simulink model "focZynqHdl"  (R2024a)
settings: Solver=FixedStepDiscrete  StartTime=0.0  StopTime=inf  RelTol=1e-3
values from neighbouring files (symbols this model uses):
  dataRange = Rotor velocity
                        radian/sec
                        800.0
                        -800.0
                    
                
                
                    
                        Phase current
                        Ampere
                        12.0
                        -12.0    [focZynqData.sldd]
  encoder = US Digital E2-1250-197-HI
                0.0
                0
                1250.0
                5000.0
                0.0012566370614359172
                0
                20.0    [focZynqData.sldd]
  paramAdcAmperePerCount = -0.000960526315789474 -0.000968421052631579
                
                    
                        Auto
                        
                        
                        -1.0
                        Simulink
                        Parameter
                        Default    [focZynqData.sldd]
  paramAdcCountAtZeroAmpere = 32600.0 32700.0
                
                    
                        Auto
                        
                        
                        -1.0
                        Simulink
                        Parameter
                        Default
                        
                            
                                0    [focZynqData.sldd]
  paramCurrentControlI = 1774.2
                
                    
                        Auto
                        
                        
                        -1.0
                        Simulink
                        Parameter
                        Default
                        
                            
                                0    [focZynqData.sldd]
  paramCurrentControlP = 1.36193
                
                    
                        Auto
                        
                        
                        -1.0
                        Simulink
                        Parameter
                        Default
                        
                            
                                0    [focZynqData.sldd]
  paramCurrentControlSatVoltage = 13.856406460551021
                
                    
                        Auto
                        
                        
                        -1.0
                        Simulink
                        Parameter
                        Default
                        
                            
                                0    [focZynqData.sldd]
  paramEncoderRotorPositionPerCount = 0.0012566370614359172
                
                    
                        Auto
                        
                        
                        -1.0
                        Simulink
                        Parameter
                        Default
                        
                            
                                0    [focZynqData.sldd]
  paramOverCurrentDuration = 0.05
                
                    
                        Auto
                        
                        
                        -1.0
                        Simulink
                        Parameter
                        Default
                        
                            
                                0    [focZynqData.sldd]
  paramOverCurrentEnable = 0.0
                
                    
                        Auto
                        
                        
                        -1.0
                        Simulink
                        Parameter
                        Default
                        
                            
                                0    [focZynqData.sldd]
  paramOverCurrentLimit = 10.45
                
                    
                        Auto
                        
                        
                        -1.0
                        Simulink
                        Parameter
                        Default
                        
                            
                                0    [focZynqData.sldd]
  paramPwmCompareAtZeroVolt = 500.0
                
                    
                        Auto
                        
                        
                        -1.0
                        Simulink
                        Parameter
                        Default
                        
                            
                                0    [focZynqData.sldd]
  paramPwmCompareMax = 1000.0
                
                    
                        Auto
                        
                        
                        -1.0
                        Simulink
                        Parameter
                        Default
                        
                            
                                0    [focZynqData.sldd]
  paramPwmComparePerVolt = 41.666666666666664
                
                    
                        Auto
                        
                        
                        -1.0
                        Simulink
                        Parameter
                        Default
                        
                            
                                0    [focZynqData.sldd]
  pmsm = Dyno 1: BLY172D-24V-4000 Anaheim Automation
                BLY172D-24V-4000 Anaheim Automation
Phase A leads B leads C for counterclockwise rotation
-----------------------------------------------------
Phase A = Yellow
Phase B = Red
Phase C = Black
                
                    
                        Watt
                        Volt
                        rad/sec    [focZynqData.sldd]
  pwm = 2.0E-8
                4.0E-5
                1000.0
                2000.0
                5.0
                1.0E-7    [focZynqData.sldd]
  sampleTime = 4.0E-5
                0.001
                0.001
                4.0E-5
                2.0E-8
                4.0E-5
                0.001
                2.0E-8
                2.0E-8
                2.0E-8    [focZynqData.sldd]
undefined symbols (not defined in the file or in its folder): hex2dec
libraries: simulink x8
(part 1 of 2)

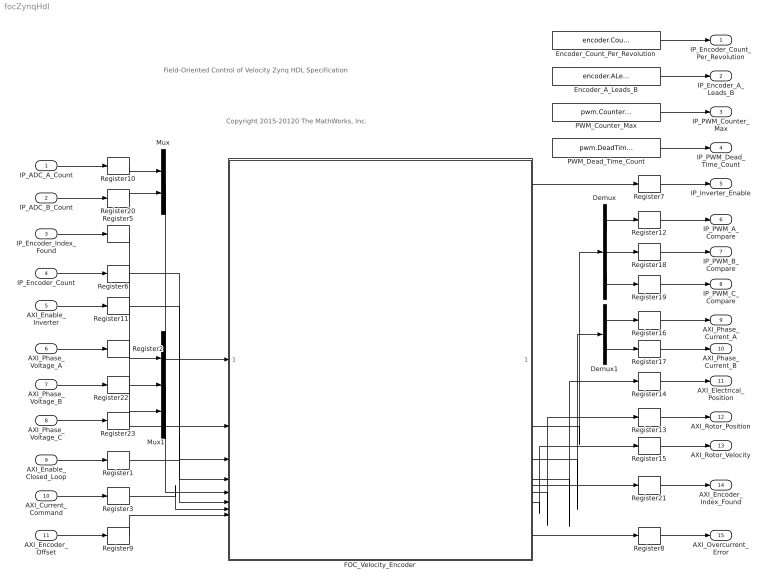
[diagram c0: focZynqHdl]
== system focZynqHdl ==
  note: Field-Oriented Control of Velocity Zynq HDL Specification
  note: Copyright 2015-20120 The MathWorks, Inc.
  IP_ADC_A_Count : Inport  PortDimensions=1  Interpolate=off
  IP_ADC_B_Count : Inport  Port=2  PortDimensions=1  Interpolate=off
  IP_Encoder_Index_Found : Inport  Port=3  Interpolate=off
  IP_Encoder_Count : Inport  Port=4  Interpolate=off
  AXI_Enable_Inverter : Inport  Port=5
  AXI_Phase_Voltage_A : Inport  Port=6
  AXI_Phase_Voltage_B : Inport  Port=7
  AXI_Phase_Voltage_C : Inport  Port=8
  AXI_Enable_Closed_Loop : Inport  Port=9
  AXI_Current_Command : Inport  Port=10
  AXI_Encoder_Offset : Inport  Port=11
  Demux : Demux  Outputs=3
  Demux1 : Demux  Outputs=2
  Encoder_A_Leads_B : Constant  Value=encoder.ALeadsB  OutDataTypeStr=fixdt(0,1,0)  SampleTime=-1
  Encoder_Count_Per_Revolution : Constant  Value=encoder.CountPerRevolution  OutDataTypeStr=fixdt(0,15,0)  SampleTime=-1
  FOC_Velocity_Encoder : Subsystem
  Mux : Mux  Inputs=2
  Mux1 : Mux  Inputs=3
  PWM_Counter_Max : Constant  Value=pwm.CounterMax  OutDataTypeStr=uint16  SampleTime=-1
  PWM_Dead_Time_Count : Constant  Value=pwm.DeadTimeCount  OutDataTypeStr=uint8  SampleTime=-1
  Register{1..3,5..23} (22 alike) : Delay  DelayLength=1
  IP_Encoder_Count_Per_Revolution : Outport  VectorParamsAs1DForOutWhenUnconnected=off
  IP_Encoder_A_Leads_B : Outport  Port=2  VectorParamsAs1DForOutWhenUnconnected=off
  IP_PWM_Counter_Max : Outport  Port=3  VectorParamsAs1DForOutWhenUnconnected=off
  IP_PWM_Dead_Time_Count : Outport  Port=4  VectorParamsAs1DForOutWhenUnconnected=off
  IP_Inverter_Enable : Outport  Port=5  VectorParamsAs1DForOutWhenUnconnected=off
  IP_PWM_A_Compare : Outport  Port=6  VectorParamsAs1DForOutWhenUnconnected=off
  IP_PWM_B_Compare : Outport  Port=7  VectorParamsAs1DForOutWhenUnconnected=off
  IP_PWM_C_Compare : Outport  Port=8  VectorParamsAs1DForOutWhenUnconnected=off
  AXI_Phase_Current_A : Outport  Port=9  VectorParamsAs1DForOutWhenUnconnected=off
  AXI_Phase_Current_B : Outport  Port=10  VectorParamsAs1DForOutWhenUnconnected=off
  AXI_Electrical_Position : Outport  Port=11  VectorParamsAs1DForOutWhenUnconnected=off
  AXI_Rotor_Position : Outport  Port=12  VectorParamsAs1DForOutWhenUnconnected=off
  AXI_Rotor_Velocity : Outport  Port=13  VectorParamsAs1DForOutWhenUnconnected=off
  AXI_Encoder_Index_Found : Outport  Port=14  VectorParamsAs1DForOutWhenUnconnected=off
  AXI_Overcurrent_Error : Outport  Port=15  VectorParamsAs1DForOutWhenUnconnected=off
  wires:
  Demux/2 -> Register18/1
  Demux/3 -> Register19/1
  Demux1/2 -> Register17/1
  IP_ADC_A_Count/1 -> Register10/1
  IP_ADC_B_Count/1 -> Register20/1
  Encoder_Count_Per_Revolution/1 -> IP_Encoder_Count_Per_Revolution/1
  Encoder_A_Leads_B/1 -> IP_Encoder_A_Leads_B/1
  Register15/1 -> AXI_Rotor_Velocity/1
  Register14/1 -> AXI_Electrical_Position/1
  Register13/1 -> AXI_Rotor_Position/1
  Register8/1 -> AXI_Overcurrent_Error/1
  Register7/1 -> IP_Inverter_Enable/1
  IP_Encoder_Count/1 -> Register6/1
  AXI_Current_Command/1 -> Register3/1
  AXI_Phase_Voltage_A/1 -> Register2/1
  AXI_Enable_Closed_Loop/1 -> Register1/1
  Demux/1 -> Register12/1
  Demux1/1 -> Register16/1
  Register16/1 -> AXI_Phase_Current_A/1
  Register17/1 -> AXI_Phase_Current_B/1
  Register12/1 -> IP_PWM_A_Compare/1
  Register18/1 -> IP_PWM_B_Compare/1
  Register19/1 -> IP_PWM_C_Compare/1
  Register10/1 -> Mux/1
  Register20/1 -> Mux/2
  Register5/1 -> FOC_Velocity_Encoder/2(Encoder_Index_Found1)
  IP_Encoder_Index_Found/1 -> Register5/1
  Register1/1 -> FOC_Velocity_Encoder/6(Enable_Current_Control1)
  Mux1/1 -> FOC_Velocity_Encoder/5(Phase_Voltage_Command)
  Register3/1 -> FOC_Velocity_Encoder/7(Current_Command)
  Mux/1 -> FOC_Velocity_Encoder/1(ADC_Phase_Currents)
  Register6/1 -> FOC_Velocity_Encoder/3(Encoder_Count)
  FOC_Velocity_Encoder/3(Phase_Currents) -> Demux1/1
  FOC_Velocity_Encoder/5(Rotor_Position) -> Register13/1
  FOC_Velocity_Encoder/4(Electrical_Position) -> Register14/1
  FOC_Velocity_Encoder/6(Rotor_Velocity) -> Register15/1
  FOC_Velocity_Encoder/2(PWM_Compare) -> Demux/1
  FOC_Velocity_Encoder/8(Error) -> Register8/1
  AXI_Encoder_Offset/1 -> Register9/1
  Register9/1 -> FOC_Velocity_Encoder/8(Encoder_Offset)
  AXI_Enable_Inverter/1 -> Register11/1
  Register11/1 -> FOC_Velocity_Encoder/4(Enable_Inverter_In)
  FOC_Velocity_Encoder/1(Enable_Inverter_Out) -> Register7/1
  Register21/1 -> AXI_Encoder_Index_Found/1
  FOC_Velocity_Encoder/7(Encoder_Index_Found_Out) -> Register21/1
  AXI_Phase_Voltage_B/1 -> Register22/1
  AXI_Phase_Voltage_C/1 -> Register23/1
  Register2/1 -> Mux1/1
  Register22/1 -> Mux1/2
  Register23/1 -> Mux1/3
  PWM_Counter_Max/1 -> IP_PWM_Counter_Max/1
  PWM_Dead_Time_Count/1 -> IP_PWM_Dead_Time_Count/1

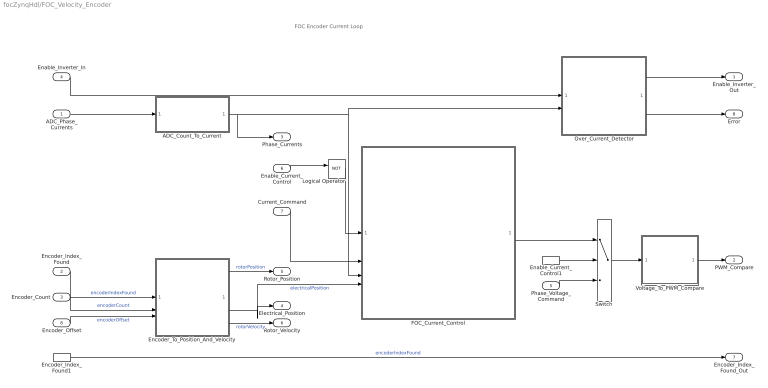
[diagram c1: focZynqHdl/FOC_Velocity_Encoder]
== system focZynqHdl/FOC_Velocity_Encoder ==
  note: FOC Encoder Current Loop
  ADC_Phase_Currents : Inport
  Encoder_Index_Found : Inport  Port=2
  Encoder_Count : Inport  Port=3
  Enable_Inverter_In : Inport  Port=4  OutDataTypeStr=boolean
  Phase_Voltage_Command : Inport  Port=5
  Enable_Current_Control : Inport  Port=6  OutMin=0  OutMax=1  OutDataTypeStr=boolean
  Current_Command : Inport  Port=7
  Encoder_Offset : Inport  Port=8
  ADC_Count_To_Current : Subsystem
  Enable_Current_Control1 : InportShadow  Port=6  OutMin=0  OutMax=1  OutDataTypeStr=boolean
  Encoder_Index_Found1 : InportShadow  Port=2
  Encoder_To_Position_And_Velocity : Subsystem  VariantControl=ctrlVariantPosSns==PosSnsEnum.Encoder
  FOC_Current_Control : Subsystem  Variant=on  VariantControlMode=label  VariantControl=Choice  LabelModeActiveChoice=Default
  Logical Operator : Logic  Operator=NOT  IconShape=distinctive  AllPortsSameDT=off  OutDataTypeStr=boolean
  Over_Current_Detector : Subsystem
  Switch : Switch  Criteria=u2 ~= 0
  Voltage_To_PWM_Compare : Subsystem
  Enable_Inverter_Out : Outport  OutMin=0  OutMax=1  VectorParamsAs1DForOutWhenUnconnected=off
  PWM_Compare : Outport  Port=2  VectorParamsAs1DForOutWhenUnconnected=off
  Phase_Currents : Outport  Port=3  VectorParamsAs1DForOutWhenUnconnected=off
  Electrical_Position : Outport  Port=4  VectorParamsAs1DForOutWhenUnconnected=off
  Rotor_Position : Outport  Port=5  VectorParamsAs1DForOutWhenUnconnected=off
  Rotor_Velocity : Outport  Port=6  VectorParamsAs1DForOutWhenUnconnected=off
  Encoder_Index_Found_Out : Outport  Port=7  OutMin=0  OutMax=1  VectorParamsAs1DForOutWhenUnconnected=off
  Error : Outport  Port=8  OutMin=0  OutMax=1  VectorParamsAs1DForOutWhenUnconnected=off
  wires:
  Encoder_To_Position_And_Velocity/2(Electrical_Position) -> Electrical_Position/1, FOC_Current_Control/4(Electrical_Position)  "electricalPosition"
  Over_Current_Detector/2(Error) -> Error/1
  ADC_Phase_Currents/1 -> ADC_Count_To_Current/1(Count)
  Encoder_Index_Found/1 -> Encoder_To_Position_And_Velocity/1(Index_Found)  "encoderIndexFound"
  Encoder_Count/1 -> Encoder_To_Position_And_Velocity/2(Count)  "encoderCount"
  Encoder_Offset/1 -> Encoder_To_Position_And_Velocity/3(Offset)  "encoderOffset"
  Phase_Voltage_Command/1 -> Switch/3
  ADC_Count_To_Current/1(Current) -> FOC_Current_Control/3(Phase_Current), Over_Current_Detector/2(Phase_Current), Phase_Currents/1
  Encoder_To_Position_And_Velocity/1(Rotor_Position) -> Rotor_Position/1  "rotorPosition"
  Encoder_To_Position_And_Velocity/3(Rotor_Velocity) -> Rotor_Velocity/1  "rotorVelocity"
  Voltage_To_PWM_Compare/1(Compare) -> PWM_Compare/1
  Switch/1 -> Voltage_To_PWM_Compare/1(Voltage)
  Enable_Current_Control/1 -> Logical Operator/1
  Enable_Current_Control1/1 -> Switch/2
  Enable_Inverter_In/1 -> Over_Current_Detector/1(Motor_On)
  Encoder_Index_Found1/1 -> Encoder_Index_Found_Out/1  "encoderIndexFound"
  Over_Current_Detector/1(En_Inv) -> Enable_Inverter_Out/1
  Logical Operator/1 -> FOC_Current_Control/1(Reset)
  Current_Command/1 -> FOC_Current_Control/2(Current_Command)
  FOC_Current_Control/1(Phase_Voltage) -> Switch/1

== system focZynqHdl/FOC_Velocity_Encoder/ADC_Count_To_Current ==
  note: ADC Count to Current
  Count : Inport  OutMin=0  OutMax=2^16-1  OutDataTypeStr=uint16
  Add : Sum  Inputs=+-  OutDataTypeStr=int16
  Bias_To_Remove : Constant  Value=paramAdcCountAtZeroAmpere  OutDataTypeStr=int16  SampleTime=-1
  Data_Type_Convert : DataTypeConversion  OutDataTypeStr=int32
  Product : Product  OutDataTypeStr=fixdt(1,32,19)
  Sat : Saturate  UpperLimit=dataRange.PhaseCurrent.Max  LowerLimit=dataRange.PhaseCurrent.Min  OutDataTypeStr=fixdt(1,16,11)
  Scalar : Constant  Value=paramAdcAmperePerCount  OutDataTypeStr=fixdt(1,16,19)  SampleTime=-1
  Current : Outport  VectorParamsAs1DForOutWhenUnconnected=off
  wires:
  Bias_To_Remove/1 -> Add/2
  Scalar/1 -> Product/2
  Add/1 -> Product/1
  Count/1 -> Data_Type_Convert/1
  Data_Type_Convert/1 -> Add/1
  Product/1 -> Sat/1
  Sat/1 -> Current/1

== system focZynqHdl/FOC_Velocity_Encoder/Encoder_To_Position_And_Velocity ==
  note: Encoder To Position And Velocity
  Index_Found : Inport
  Count : Inport  Port=2  SampleTime=sampleTime.EncoderPosition
  Offset : Inport  Port=3  SampleTime=sampleTime.EncoderPosition
  Encoder_Count_To_Rotor_Position1 : Subsystem
  Rotor_Position_Delta : Subsystem
  Rotor_Position_Delta_To_Velocity : Subsystem  mask(Rotor position delta to velocity){positionDeltaBufferLength=32, sampleFrequency=1/sampleTime.EncoderPosition}
      mask prompts: positionDeltaBufferLength "Delay buffer length (must be power of two)"; sampleFrequency "Sample frequency (Hz)"
      mask help: Calculates velocity by summing the current position delta and a buffer of previous position deltas. Previous position deltas are stored in a circular buffer.
  Rotor_To_Electrical_Position_No_Overflow_Fixpt : Subsystem
  Rotor_Position : Outport  VectorParamsAs1DForOutWhenUnconnected=off
  Electrical_Position : Outport  Port=2  VectorParamsAs1DForOutWhenUnconnected=off
  Rotor_Velocity : Outport  Port=3  VectorParamsAs1DForOutWhenUnconnected=off
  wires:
  Rotor_Position_Delta/1(Position_Delta) -> Rotor_Position_Delta_To_Velocity/1(Position_Delta)  "rotorPositionDelta"
  Rotor_To_Electrical_Position_No_Overflow_Fixpt/1(E) -> Electrical_Position/1
  Count/1 -> Encoder_Count_To_Rotor_Position1/1(Count)
  Index_Found/1 -> Rotor_Position_Delta/3(Encoder_Index_Found)
  Rotor_Position_Delta_To_Velocity/1(Velocity) -> Rotor_Velocity/1
  Encoder_Count_To_Rotor_Position1/1(Position) -> Rotor_Position_Delta/1(Rotor_Position), Rotor_To_Electrical_Position_No_Overflow_Fixpt/1(R), Rotor_Position/1
  Offset/1 -> Rotor_Position_Delta/2(Encoder_Offset), Encoder_Count_To_Rotor_Position1/2(Position_At_Zero_Count)

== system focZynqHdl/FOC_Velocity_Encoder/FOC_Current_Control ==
  Reset : Inport
  Current_Command : Inport  Port=2  OutDataTypeStr=fixdt(1,16,11)
  Phase_Current : Inport  Port=3
  Electrical_Position : Inport  Port=4
  FOC_Current_Control : Subsystem  VariantControl=Default
  FloatingPoint_FOC_Control : Subsystem  VariantControl=Alternative
  Phase_Voltage : Outport

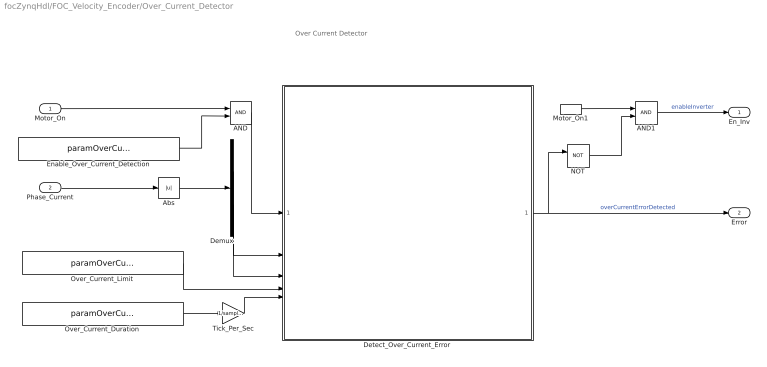
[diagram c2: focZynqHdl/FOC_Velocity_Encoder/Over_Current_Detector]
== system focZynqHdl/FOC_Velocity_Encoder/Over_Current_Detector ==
  note: Over Current Detector
  Motor_On : Inport  OutMin=0  OutMax=1  OutDataTypeStr=boolean
  Phase_Current : Inport  Port=2  OutMin=dataRange.PhaseCurrent.Min  OutMax=dataRange.PhaseCurrent.Max  OutDataTypeStr=fixdt(1,16,11)
  AND : Logic  IconShape=distinctive  AllPortsSameDT=off  OutDataTypeStr=boolean
  AND1 : Logic  IconShape=distinctive  AllPortsSameDT=off  OutDataTypeStr=boolean
  Abs : Abs
  Demux : Demux  Outputs=2
  Detect_Over_Current_Error : Stateflow chart  TreatAsAtomicUnit=on
  Enable_Over_Current_Detection : Constant  Value=paramOverCurrentEnable  OutDataTypeStr=boolean  SampleTime=-1
  Motor_On1 : InportShadow  OutMin=0  OutMax=1  OutDataTypeStr=boolean
  NOT : Logic  Operator=NOT  IconShape=distinctive  AllPortsSameDT=off  OutDataTypeStr=boolean
  Over_Current_Duration : Constant  Value=paramOverCurrentDuration  OutDataTypeStr=fixdt(1,16,14)  SampleTime=-1
  Over_Current_Limit : Constant  Value=paramOverCurrentLimit  OutDataTypeStr=fixdt(1,16,11)  SampleTime=-1
  Tick_Per_Sec : Gain  Gain=1/sampleTime.OverCurrentDetector  ParamDataTypeStr=fixdt(1,16,0)  OutDataTypeStr=uint16
  En_Inv : Outport  VectorParamsAs1DForOutWhenUnconnected=off
  Error : Outport  Port=2  VectorParamsAs1DForOutWhenUnconnected=off
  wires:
  Tick_Per_Sec/1 -> Detect_Over_Current_Error/5(overCurrentDurationTicks)
  Phase_Current/1 -> Abs/1
  Abs/1 -> Demux/1
  Demux/2 -> Detect_Over_Current_Error/3(phaseCurrentB)
  Detect_Over_Current_Error/1(error) -> Error/1, NOT/1  "overCurrentErrorDetected"
  Over_Current_Duration/1 -> Tick_Per_Sec/1
  Over_Current_Limit/1 -> Detect_Over_Current_Error/4(overCurrentLimit)
  Demux/1 -> Detect_Over_Current_Error/2(phaseCurrentA)
  Motor_On/1 -> AND/1
  AND1/1 -> En_Inv/1  "enableInverter"
  NOT/1 -> AND1/2
  Motor_On1/1 -> AND1/1
  AND/1 -> Detect_Over_Current_Error/1(enableOverCurrentDetect)
  Enable_Over_Current_Detection/1 -> AND/2

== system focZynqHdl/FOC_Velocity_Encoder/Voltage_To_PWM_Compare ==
  note: Voltage To PWM Compare
  Voltage : Inport  OutMin=dataRange.PhaseVoltage.Min  OutMax=dataRange.PhaseVoltage.Max  OutDataTypeStr=fixdt(1,16,11)
  Add : Sum  OutDataTypeStr=fixdt(1,32,17)
  Bias : Constant  Value=paramPwmCompareAtZeroVolt  OutDataTypeStr=fixdt(1,16,2)  SampleTime=-1
  Data_Type_Conversion : DataTypeConversion  OutDataTypeStr=uint16
  Saturation : Saturate  UpperLimit=paramPwmCompareMax  LowerLimit=0
  Slope : Gain  Gain=paramPwmComparePerVolt  ParamDataTypeStr=fixdt(1,16,6)  OutDataTypeStr=fixdt(1,32,18)
  Compare : Outport  VectorParamsAs1DForOutWhenUnconnected=off
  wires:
  Data_Type_Conversion/1 -> Compare/1  "pwmCompare"
  Voltage/1 -> Slope/1  "phaseVoltage"
  Slope/1 -> Add/1
  Saturation/1 -> Data_Type_Conversion/1
  Bias/1 -> Add/2
  Add/1 -> Saturation/1

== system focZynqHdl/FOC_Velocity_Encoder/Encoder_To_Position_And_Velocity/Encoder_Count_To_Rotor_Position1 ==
  note: Encoder Count To Rotor Position
  Count : Inport  OutMin=dataRange.EncoderCount.Min  OutMax=dataRange.EncoderCount.Max  OutDataTypeStr=fixdt(0,16,0)
  Position_At_Zero_Count : Inport  Port=2  OutMin=-2*pi  OutMax=2*pi  OutDataTypeStr=fixdt(1,16,12)
  Add : Sum  OutDataTypeStr=fixdt(1,32,27)
  Data_Type_Convert : DataTypeConversion  OutDataTypeStr=fixdt(1,16,12)  RndMeth=Simplest
  Mod_Two_Pi_Once : Subsystem
  Rotor_Position_Per_Count : Gain  Gain=paramEncoderRotorPositionPerCount  ParamDataTypeStr=fixdt(1,16,22)  OutDataTypeStr=fixdt(1,32,25)
  Position : Outport  VectorParamsAs1DForOutWhenUnconnected=off
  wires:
  Count/1 -> Rotor_Position_Per_Count/1
  Position_At_Zero_Count/1 -> Add/2
  Rotor_Position_Per_Count/1 -> Add/1
  Add/1 -> Mod_Two_Pi_Once/1(X)
  Mod_Two_Pi_Once/1(Mod_X_Two_Pi) -> Data_Type_Convert/1  "rotorPosition"
  Data_Type_Convert/1 -> Position/1

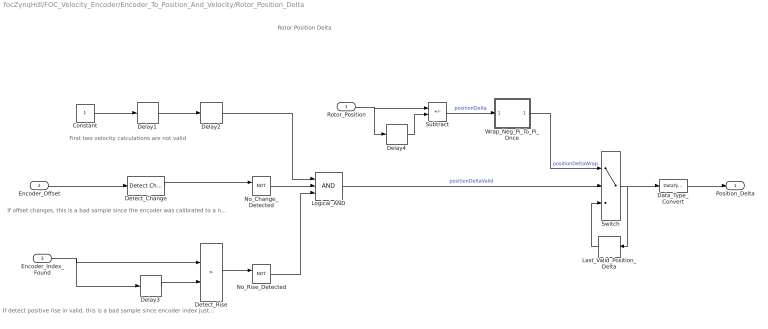
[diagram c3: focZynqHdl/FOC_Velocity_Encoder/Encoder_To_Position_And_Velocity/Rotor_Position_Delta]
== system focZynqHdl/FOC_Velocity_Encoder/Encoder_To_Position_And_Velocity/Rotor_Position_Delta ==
  note: Rotor Position Delta
  note: If detect positive rise in valid, this is a bad sample since encoder index just reset
  note: First two velocity calculations are not valid
  note: If offset changes, this is a bad sample since the encoder was calibrated to a new value
  Rotor_Position : Inport  OutMin=0  OutMax=2*pi  OutDataTypeStr=fixdt(1,16,12)  SampleTime=sampleTime.EncoderPosition
  Encoder_Offset : Inport  Port=2  OutMin=-2*pi  OutMax=2*pi  OutDataTypeStr=fixdt(1,16,12)  SampleTime=sampleTime.EncoderPosition
  Encoder_Index_Found : Inport  Port=3  OutDataTypeStr=boolean  SampleTime=sampleTime.EncoderPosition
  Constant : Constant  OutDataTypeStr=fixdt(1,16,14)  SampleTime=-1
  Data_Type_Convert : DataTypeConversion  OutDataTypeStr=fixdt(1,16,13)  RndMeth=Simplest
  Delay{1..4} (4 alike) : Delay  DelayLength=1
  Detect_Change : simulink/Logic and Bit Operations/Detect Change  vinit=0  OutDataTypeStr=boolean
  Detect_Rise : RelationalOperator  Operator=>  OutDataTypeStr=boolean  ZeroCross=off
  Last_Valid_Position_Delta : Delay  DelayLength=1
  Logical_AND : Logic  Inputs=3  IconShape=distinctive  AllPortsSameDT=off  OutDataTypeStr=boolean
  No_Change_Detected : Logic  Operator=NOT  IconShape=distinctive  AllPortsSameDT=off  OutDataTypeStr=boolean
  No_Rise_Detected : Logic  Operator=NOT  IconShape=distinctive  AllPortsSameDT=off  OutDataTypeStr=boolean
  Subtract : Sum  Inputs=+-  OutDataTypeStr=fixdt(1,32,27)  InputSameDT=on
  Switch : Switch  Criteria=u2 ~= 0  OutDataTypeStr=fixdt(1,32,29)
  Wrap_Neg_Pi_To_Pi_Once : Subsystem
  Position_Delta : Outport  SampleTime=sampleTime.EncoderPosition  VectorParamsAs1DForOutWhenUnconnected=off
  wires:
  Delay1/1 -> Delay2/1
  Constant/1 -> Delay1/1
  Switch/1 -> Last_Valid_Position_Delta/1, Data_Type_Convert/1
  No_Rise_Detected/1 -> Logical_AND/3
  Detect_Rise/1 -> No_Rise_Detected/1
  Last_Valid_Position_Delta/1 -> Switch/3
  Delay3/1 -> Detect_Rise/2
  Logical_AND/1 -> Switch/2  "positionDeltaValid"
  Delay4/1 -> Subtract/2
  Delay2/1 -> Logical_AND/1
  Subtract/1 -> Wrap_Neg_Pi_To_Pi_Once/1(Position)  "positionDelta"
  Rotor_Position/1 -> Delay4/1, Subtract/1
  Encoder_Index_Found/1 -> Delay3/1, Detect_Rise/1
  Wrap_Neg_Pi_To_Pi_Once/1(Wrap) -> Switch/1  "positionDeltaWrap"
  Encoder_Offset/1 -> Detect_Change/1
  Detect_Change/1 -> No_Change_Detected/1
  No_Change_Detected/1 -> Logical_AND/2
  Data_Type_Convert/1 -> Position_Delta/1

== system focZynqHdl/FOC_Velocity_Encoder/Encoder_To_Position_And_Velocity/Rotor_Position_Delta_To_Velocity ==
  note: Rotor Position Delta To Velocity
  Position_Delta : Inport  OutMin=-pi  OutMax=pi  OutDataTypeStr=fixdt(1,16,13)  SampleTime=sampleTime.EncoderPosition
  Rotor_Position_Delta_To_Velocity : MATLAB Function  TreatAsAtomicUnit=on
  Velocity : Outport  SampleTime=sampleTime.EncoderPosition  VectorParamsAs1DForOutWhenUnconnected=off
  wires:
  Position_Delta/1 -> Rotor_Position_Delta_To_Velocity/1(positionDelta)
  Rotor_Position_Delta_To_Velocity/1(rotorVelocity) -> Velocity/1

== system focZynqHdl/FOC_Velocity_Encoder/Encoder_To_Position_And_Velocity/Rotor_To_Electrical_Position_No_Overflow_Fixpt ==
  note: Rotor To Electrical Position
  note: Fixed-point implementation which avoids overflow
  R : Inport  OutDataTypeStr=fixdt(1,16,12)
  Extract_Lower_Bits1 : simulink/Logic and Bit Operations/Bitwise Operator  logicop=AND  UseBitMask=on  BitMask=hex2dec('FFFF')  BitMaskRealWorld=Stored Integer
  Extract_Lower_Bits2 : simulink/Logic and Bit Operations/Bitwise Operator  logicop=AND  UseBitMask=on  BitMask=hex2dec('FFFF')  BitMaskRealWorld=Stored Integer
  Input_Range : SignalSpecification  OutMin=0  OutMax=2*pi
  Normalize : Gain  Gain=1/(2*pi)  ParamDataTypeStr=fixdt(0,16,18)  OutDataTypeStr=fixdt(0,32,16, 'DataTypeOverride', 'Off')
  Pole_Pair_Gain : Gain  Gain=pmsm.PolePairs  ParamDataTypeStr=uint16  OutDataTypeStr=fixdt('uint32', 'DataTypeOverride', 'Off')
  Scale_To_Two_Pi : Gain  Gain=2*pi  ParamDataTypeStr=fixdt(0,16,13)  OutDataTypeStr=fixdt(0,16,12)
  Signed_Fixpt : DataTypeConversion  OutDataTypeStr=fixdt(1,16,12)  ConvertRealWorld=Stored Integer (SI)
  Unsigned_Fixpt : DataTypeConversion  OutDataTypeStr=fixdt(0,16,16, 'DataTypeOverride', 'Off')  ConvertRealWorld=Stored Integer (SI)
  Unsigned_Integer : DataTypeConversion  OutDataTypeStr=fixdt('uint16', 'DataTypeOverride', 'Off')  ConvertRealWorld=Stored Integer (SI)
  E : Outport  VectorParamsAs1DForOutWhenUnconnected=off
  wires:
  R/1 -> Input_Range/1
  Unsigned_Integer/1 -> Pole_Pair_Gain/1
  Pole_Pair_Gain/1 -> Extract_Lower_Bits2/1
  Normalize/1 -> Extract_Lower_Bits1/1
  Extract_Lower_Bits2/1 -> Unsigned_Fixpt/1
  Scale_To_Two_Pi/1 -> Signed_Fixpt/1
  Unsigned_Fixpt/1 -> Scale_To_Two_Pi/1
  Signed_Fixpt/1 -> E/1
  Input_Range/1 -> Normalize/1
  Extract_Lower_Bits1/1 -> Unsigned_Integer/1

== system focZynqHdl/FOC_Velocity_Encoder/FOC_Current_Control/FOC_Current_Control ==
  note: FOC Current Control
  Reset : Inport  SampleTime=sampleTime.CurrentControl
  Current_Command : Inport  Port=2  OutMin=dataRange.PhaseCurrent.Min  OutMax=dataRange.PhaseCurrent.Max  OutDataTypeStr=fixdt(1,16,11)  SampleTime=sampleTime.CurrentControl
  Phase_Current : Inport  Port=3  OutMin=dataRange.PhaseCurrent.Min  OutMax=dataRange.PhaseCurrent.Max  OutDataTypeStr=fixdt(1,16,11)  SampleTime=sampleTime.CurrentControl
  Electrical_Position : Inport  Port=4  OutMin=0  OutMax=2*pi  OutDataTypeStr=fixdt(1,16,12)  SampleTime=sampleTime.CurrentControl
  Clarke_Transform : Subsystem
  DQ_Current_Control : Subsystem
  Inverse_Clarke_Transform : Subsystem  VariantControl=INVERSE_CLARKE_TRANSFORM
  Inverse_Park_Transform : Subsystem
  Park_Transform : Subsystem
  Sat : Saturate  UpperLimit=dataRange.PhaseVoltage.Max  LowerLimit=dataRange.PhaseVoltage.Min  OutDataTypeStr=fixdt(1,16,11)
  Sine_Cosine : Subsystem
  Space_Vector_Modulation : Subsystem  VariantControl=SpaceVectorModulation_JB
  Phase_Voltage : Outport  SampleTime=sampleTime.CurrentControl  VectorParamsAs1DForOutWhenUnconnected=off
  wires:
  Sine_Cosine/1(Sin) -> Park_Transform/3(Sin_Coefficient1), Inverse_Park_Transform/3(Sin_Coefficient1)  "sinCoefficient"
  Sine_Cosine/2(Cos) -> Park_Transform/4(Cos_Coefficient1), Inverse_Park_Transform/4(Cos_Coefficient1)  "cosCoefficient"
  Inverse_Clarke_Transform/1(ABC) -> Space_Vector_Modulation/1(ABC)  "abcVoltage"
  Electrical_Position/1 -> Sine_Cosine/1(P)
  Phase_Current/1 -> Clarke_Transform/1(ABC)
  Clarke_Transform/1(Alpha) -> Park_Transform/1(Alpha)  "alphaCurrent"
  Clarke_Transform/2(Beta) -> Park_Transform/2(Beta1)  "betaCurrent"
  Inverse_Park_Transform/1(Alpha) -> Inverse_Clarke_Transform/1(Alpha)  "alphaVoltage"
  Inverse_Park_Transform/2(Beta) -> Inverse_Clarke_Transform/2(Beta)  "betaVoltage"
  Park_Transform/1(D) -> DQ_Current_Control/3(D_Current)  "dCurrent"
  Park_Transform/2(Q) -> DQ_Current_Control/4(Q_Current)  "qCurrent"
  Current_Command/1 -> DQ_Current_Control/2(Q_Command)
  DQ_Current_Control/1(D_Voltage) -> Inverse_Park_Transform/1(D)  "dVoltage"
  DQ_Current_Control/2(Q_Voltage) -> Inverse_Park_Transform/2(Q)  "qVoltage"
  Space_Vector_Modulation/1(ABC_SVM) -> Sat/1  "svmVoltage"
  Sat/1 -> Phase_Voltage/1
  Reset/1 -> DQ_Current_Control/1(Reset)

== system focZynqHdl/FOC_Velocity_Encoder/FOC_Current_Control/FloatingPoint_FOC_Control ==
  note: FOC Encoder Current Loop current control floating-point algorithm
  Reset : Inport
  Current_Command : Inport  Port=2
  Phase_Current : Inport  Port=3
  Electrical_Position : Inport  Port=4
  Data Type Conversion1 : DataTypeConversion  OutDataTypeStr=single  RndMeth=Nearest
  Data Type Conversion2 : DataTypeConversion  OutDataTypeStr=single  RndMeth=Nearest
  Data Type Conversion3 : DataTypeConversion  OutDataTypeStr=single  RndMeth=Nearest
  Data Type Conversion4 : DataTypeConversion  OutDataTypeStr=fixdt(1,16,11)  RndMeth=Nearest
  FOC_Current_Control : Subsystem
  Phase_Voltage : Outport  VectorParamsAs1DForOutWhenUnconnected=off
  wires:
  Current_Command/1 -> Data Type Conversion1/1
  Data Type Conversion3/1 -> FOC_Current_Control/4(Electrical_Position)
  FOC_Current_Control/1(Phase_Voltage) -> Data Type Conversion4/1
  Reset/1 -> FOC_Current_Control/1(Reset)
  Data Type Conversion1/1 -> FOC_Current_Control/2(Current_Command)
  Data Type Conversion2/1 -> FOC_Current_Control/3(Phase_Current)
  Electrical_Position/1 -> Data Type Conversion3/1
  Phase_Current/1 -> Data Type Conversion2/1
  Data Type Conversion4/1 -> Phase_Voltage/1

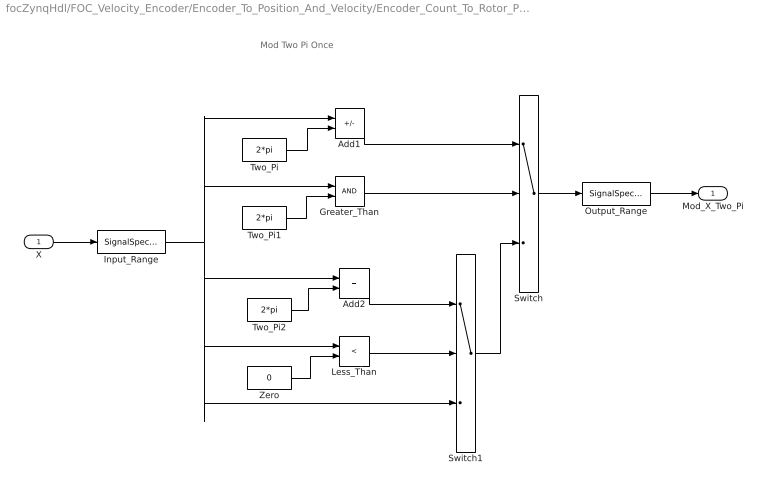
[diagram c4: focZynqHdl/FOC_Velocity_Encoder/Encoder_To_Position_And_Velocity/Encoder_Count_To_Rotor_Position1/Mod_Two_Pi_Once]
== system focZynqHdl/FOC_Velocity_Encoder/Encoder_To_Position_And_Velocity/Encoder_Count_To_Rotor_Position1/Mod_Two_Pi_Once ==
  note: Mod Two Pi Once
  X : Inport
  Add1 : Sum  Inputs=+-  OutDataTypeStr=fixdt(1,32,28)
  Add2 : Sum  OutDataTypeStr=fixdt(1,32,27)
  Greater_Than : RelationalOperator  OutDataTypeStr=boolean
  Input_Range : SignalSpecification  OutMin=-4*pi  OutMax=4*pi
  Less_Than : RelationalOperator  Operator=<  OutDataTypeStr=boolean
  Output_Range : SignalSpecification  OutMin=0  OutMax=2*pi
  Switch : Switch  Criteria=u2 ~= 0  OutDataTypeStr=fixdt(1,32,28)
  Switch1 : Switch  Criteria=u2 ~= 0  OutDataTypeStr=fixdt(1,32,28)
  Two_Pi : Constant  Value=2*pi  OutDataTypeStr=fixdt(1,16,12)  SampleTime=-1
  Two_Pi1 : Constant  Value=2*pi  OutDataTypeStr=fixdt(1,16,12)  SampleTime=-1
  Two_Pi2 : Constant  Value=2*pi  OutDataTypeStr=fixdt(1,16,12)  SampleTime=-1
  Zero : Constant  Value=0  OutDataTypeStr=fixdt(1,16,0)  SampleTime=-1
  Mod_X_Two_Pi : Outport  VectorParamsAs1DForOutWhenUnconnected=off
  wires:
  Input_Range/1 -> Switch1/3, Less_Than/1, Add2/1, Greater_Than/1, Add1/1
  Switch/1 -> Output_Range/1
  X/1 -> Input_Range/1
  Greater_Than/1 -> Switch/2
  Add1/1 -> Switch/1
  Two_Pi/1 -> Add1/2
  Two_Pi1/1 -> Greater_Than/2
  Switch1/1 -> Switch/3
  Less_Than/1 -> Switch1/2
  Add2/1 -> Switch1/1
  Two_Pi2/1 -> Add2/2
  Zero/1 -> Less_Than/2
  Output_Range/1 -> Mod_X_Two_Pi/1

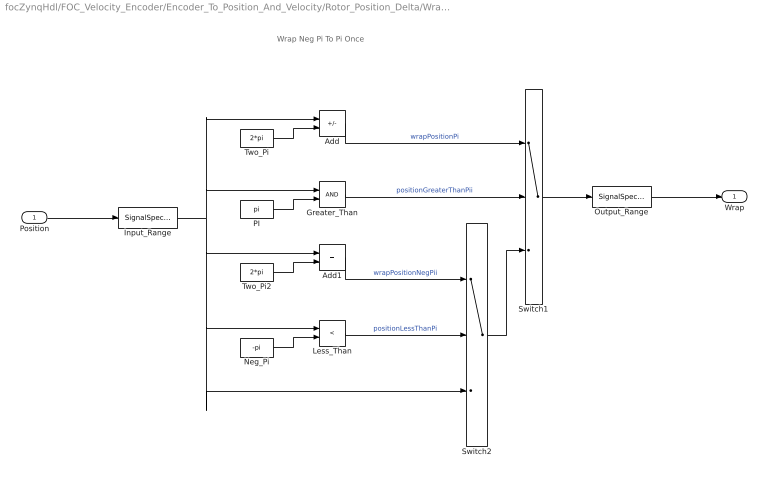
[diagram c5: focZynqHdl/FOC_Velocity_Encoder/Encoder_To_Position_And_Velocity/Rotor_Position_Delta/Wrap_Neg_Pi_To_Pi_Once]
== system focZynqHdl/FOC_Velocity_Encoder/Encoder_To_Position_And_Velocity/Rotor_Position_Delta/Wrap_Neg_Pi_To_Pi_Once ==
  note: Wrap Neg Pi To Pi Once
  Position : Inport
  Add : Sum  Inputs=+-  OutDataTypeStr=fixdt(1,32,29)
  Add1 : Sum  OutDataTypeStr=fixdt(1,32,29)
  Greater_Than : RelationalOperator  OutDataTypeStr=boolean
  Input_Range : SignalSpecification  OutMin=-4*pi  OutMax=4*pi
  Less_Than : RelationalOperator  Operator=<  OutDataTypeStr=boolean
  Neg_Pi : Constant  Value=-pi  OutDataTypeStr=fixdt(1,16,13)  SampleTime=-1
  Output_Range : SignalSpecification  OutMin=-pi  OutMax=pi
  PI : Constant  Value=pi  OutDataTypeStr=fixdt(1,16,13)  SampleTime=-1
  Switch1 : Switch  Criteria=u2 ~= 0  OutDataTypeStr=fixdt(1,32,29)
  Switch2 : Switch  Criteria=u2 ~= 0  OutDataTypeStr=fixdt(1,32,29)
  Two_Pi : Constant  Value=2*pi  OutDataTypeStr=fixdt(1,16,12)  SampleTime=-1
  Two_Pi2 : Constant  Value=2*pi  OutDataTypeStr=fixdt(1,16,12)  SampleTime=-1
  Wrap : Outport  VectorParamsAs1DForOutWhenUnconnected=off
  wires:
  Position/1 -> Input_Range/1
  PI/1 -> Greater_Than/2
  Neg_Pi/1 -> Less_Than/2
  Greater_Than/1 -> Switch1/2  "positionGreaterThanPii"
  Two_Pi/1 -> Add/2
  Add/1 -> Switch1/1  "wrapPositionPi"
  Less_Than/1 -> Switch2/2  "positionLessThanPi"
  Switch2/1 -> Switch1/3
  Two_Pi2/1 -> Add1/2
  Add1/1 -> Switch2/1  "wrapPositionNegPii"
  Switch1/1 -> Output_Range/1
  Output_Range/1 -> Wrap/1
  Input_Range/1 -> Less_Than/1, Switch2/3, Add1/1, Add/1, Greater_Than/1

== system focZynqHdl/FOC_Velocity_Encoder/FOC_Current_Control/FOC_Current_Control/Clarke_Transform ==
  note: Clarke Transform
  note: Converts balanced three-phase quantities into balanced two-phase quantities. The A and B phases are converted to the direct axis (alpha) component and the quadrature axis (beta) component. The alpha and beta components are still dependent on time and speed.
  ABC : Inport
  A : Selector  IndexMode=Zero-based  InputPortWidth=2  IndexOptions=Index vector (dialog)  Indices=0  OutputSizes=1
  Add : Sum  OutDataTypeStr=fixdt(1,16,10)
  Alpha_Gain : Gain  Gain=1/sqrt(3)  ParamDataTypeStr=fixdt(1,16,15)  OutDataTypeStr=fixdt(1,32,28)
  B : Selector  IndexMode=Zero-based  InputPortWidth=2  IndexOptions=Index vector (dialog)  Indices=1  OutputSizes=1
  Beta_Gain : Gain  Gain=2/sqrt(3)  ParamDataTypeStr=fixdt(1,16,14)  OutDataTypeStr=fixdt(1,32,27)
  Alpha : Outport  VectorParamsAs1DForOutWhenUnconnected=off
  Beta : Outport  Port=2  VectorParamsAs1DForOutWhenUnconnected=off
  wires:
  Add/1 -> Beta/1
  B/1 -> Beta_Gain/1
  Beta_Gain/1 -> Add/2
  ABC/1 -> A/1, B/1
  Alpha_Gain/1 -> Add/1
  A/1 -> Alpha_Gain/1, Alpha/1

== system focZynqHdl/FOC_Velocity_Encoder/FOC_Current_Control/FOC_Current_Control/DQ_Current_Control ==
  note: DQ Current Control
  Reset : Inport
  Q_Command : Inport  Port=2  SampleTime=sampleTime.CurrentControl
  D_Current : Inport  Port=3
  Q_Current : Inport  Port=4
  D_Command : Constant  Value=0  OutDataTypeStr=fixdt(1,16,0)  SampleTime=-1
  D_Current_Control : Subsystem
  Q_Current_Control : Subsystem
  Reset1 : InportShadow
  D_Voltage : Outport  VectorParamsAs1DForOutWhenUnconnected=off
  Q_Voltage : Outport  Port=2  VectorParamsAs1DForOutWhenUnconnected=off
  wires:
  Q_Current_Control/1(Voltage) -> Q_Voltage/1
  D_Current_Control/1(Voltage) -> D_Voltage/1
  D_Command/1 -> D_Current_Control/2(Current_Command)
  Q_Command/1 -> Q_Current_Control/2(Current_Command)
  Q_Current/1 -> Q_Current_Control/3(Current_Measured)
  D_Current/1 -> D_Current_Control/3(Current_Measured)
  Reset/1 -> D_Current_Control/1(Reset)
  Reset1/1 -> Q_Current_Control/1(Reset)

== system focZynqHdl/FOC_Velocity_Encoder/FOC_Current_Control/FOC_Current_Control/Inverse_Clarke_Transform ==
  note: Inverse Clarke Transform
  note: Converts direct axis (alpha) component and the quadrature axis (beta) component to balanced three-phase quantities The alpha and beta components are dependent on time and speed.
  Alpha : Inport
  Beta : Inport  Port=2
  Add : Sum  Inputs=-+  OutDataTypeStr=fixdt(1,32,25)
  Add1 : Sum  Inputs=--  OutDataTypeStr=fixdt(1,32,25)
  Data_Type_Convert : DataTypeConversion  OutDataTypeStr=fixdt(1,32,25)  RndMeth=Simplest
  Gain : Gain  Gain=1/2  ParamDataTypeStr=fixdt(1,16,15)  OutDataTypeStr=fixdt(1,32,27)
  Gain1 : Gain  Gain=sqrt(3)/2  ParamDataTypeStr=fixdt(1,16,15)  OutDataTypeStr=fixdt(1,32,26)
  Mux : Mux  Inputs=3
  ABC : Outport  VectorParamsAs1DForOutWhenUnconnected=off
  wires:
  Gain/1 -> Add1/1, Add/1
  Gain1/1 -> Add1/2, Add/2
  Add/1 -> Mux/2
  Add1/1 -> Mux/3
  Beta/1 -> Gain1/1
  Alpha/1 -> Gain/1, Data_Type_Convert/1
  Mux/1 -> ABC/1
  Data_Type_Convert/1 -> Mux/1

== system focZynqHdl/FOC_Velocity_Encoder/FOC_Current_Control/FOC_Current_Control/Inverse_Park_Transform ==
  note: Inverse Park Transform
  note: Converts orthogonal rotating reference frame (dq) to two-phase orthogonal stationary reference frame (alpha, beta)
  D : Inport
  Q : Inport  Port=2
  Sin_Coefficient : Inport  Port=3
  Cos_Coefficient : Inport  Port=4
  Add1 : Sum  Inputs=+-  OutDataTypeStr=fixdt(1,16,10)
  Add2 : Sum  OutDataTypeStr=fixdt(1,16,10)
  Cos_Coefficient1 : InportShadow  Port=4
  Product{1..4} (4 alike) : Product  OutDataTypeStr=fixdt(1,32,27)  RndMeth=Simplest
  Sin_Coefficient1 : InportShadow  Port=3
  Alpha : Outport  VectorParamsAs1DForOutWhenUnconnected=off
  Beta : Outport  Port=2  VectorParamsAs1DForOutWhenUnconnected=off
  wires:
  Add2/1 -> Beta/1
  Add1/1 -> Alpha/1
  Product3/1 -> Add2/1
  Product4/1 -> Add2/2
  Product1/1 -> Add1/1
  Product2/1 -> Add1/2
  Cos_Coefficient1/1 -> Product4/2
  Sin_Coefficient/1 -> Product2/2
  D/1 -> Product3/1, Product1/1
  Q/1 -> Product2/1, Product4/1
  Sin_Coefficient1/1 -> Product3/2
  Cos_Coefficient/1 -> Product1/2

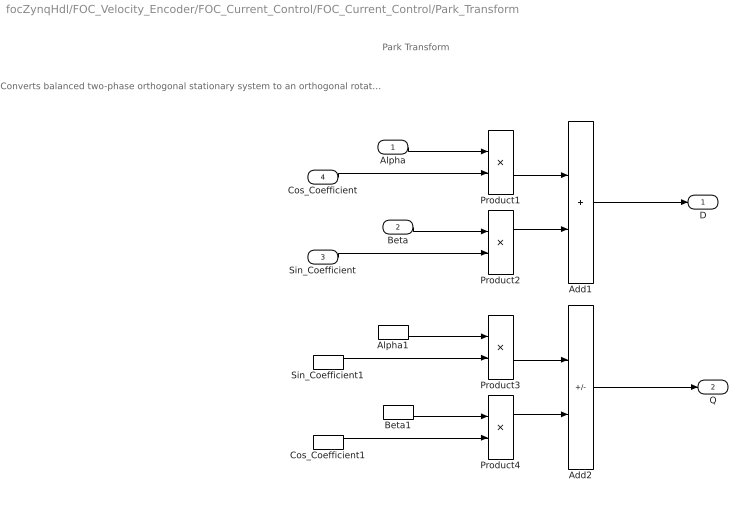
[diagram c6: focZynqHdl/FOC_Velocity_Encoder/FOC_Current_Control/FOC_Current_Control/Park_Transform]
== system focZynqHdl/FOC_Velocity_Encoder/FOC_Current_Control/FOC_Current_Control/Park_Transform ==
  note: Park Transform
  note: Converts balanced two-phase orthogonal stationary system to an orthogonal rotating reference frame.
  Alpha : Inport
  Beta : Inport  Port=2
  Sin_Coefficient : Inport  Port=3
  Cos_Coefficient : Inport  Port=4
  Add1 : Sum  OutDataTypeStr=fixdt(1,32,25)
  Add2 : Sum  Inputs=-+  OutDataTypeStr=fixdt(1,32,25)
  Alpha1 : InportShadow
  Beta1 : InportShadow  Port=2
  Cos_Coefficient1 : InportShadow  Port=4
  Product1 : Product  OutDataTypeStr=fixdt(1,32,27)  RndMeth=Simplest
  Product2 : Product  OutDataTypeStr=fixdt(1,32,26)  RndMeth=Simplest
  Product3 : Product  OutDataTypeStr=fixdt(1,32,27)  RndMeth=Simplest
  Product4 : Product  OutDataTypeStr=fixdt(1,32,26)  RndMeth=Simplest
  Sin_Coefficient1 : InportShadow  Port=3
  D : Outport  VectorParamsAs1DForOutWhenUnconnected=off
  Q : Outport  Port=2  VectorParamsAs1DForOutWhenUnconnected=off
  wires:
  Product3/1 -> Add2/1
  Product4/1 -> Add2/2
  Product1/1 -> Add1/1
  Product2/1 -> Add1/2
  Alpha1/1 -> Product3/1
  Sin_Coefficient1/1 -> Product3/2
  Cos_Coefficient1/1 -> Product4/2
  Beta1/1 -> Product4/1
  Alpha/1 -> Product1/1
  Cos_Coefficient/1 -> Product1/2
  Beta/1 -> Product2/1
  Sin_Coefficient/1 -> Product2/2
  Add1/1 -> D/1
  Add2/1 -> Q/1

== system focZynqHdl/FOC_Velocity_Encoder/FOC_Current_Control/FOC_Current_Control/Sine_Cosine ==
  note: Sine Cosine Fixed Point LUT
  P : Inport
  Normalize_Position : Gain  Gain=1/(2*pi)  ParamDataTypeStr=fixdt(1,16,17)  OutMin=0  OutMax=1  OutDataTypeStr=fixdt(1,32,30)
  Sine_Cosine_LUT : simulink/Lookup Tables/Sine  Formula=sin(2*pi*u) and cos(2*pi*u)  NumDataPoints=(2^5)+1  OutputWordLength=16  InternalRulePriority=Speed
  Sin : Outport  VectorParamsAs1DForOutWhenUnconnected=off
  Cos : Outport  Port=2  VectorParamsAs1DForOutWhenUnconnected=off
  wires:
  Sine_Cosine_LUT/2 -> Cos/1
  Sine_Cosine_LUT/1 -> Sin/1
  Normalize_Position/1 -> Sine_Cosine_LUT/1
  P/1 -> Normalize_Position/1  "position"

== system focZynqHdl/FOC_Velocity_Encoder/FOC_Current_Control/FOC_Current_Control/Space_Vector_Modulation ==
  note: Space Vector Modulation
  ABC : Inport
  Add : Sum  OutDataTypeStr=fixdt(1,16,8)
  Add1 : Sum  Inputs=+-  OutDataTypeStr=fixdt(1,32,24)
  Gain : Gain  Gain=0.5  ParamDataTypeStr=fixdt(1,16,15)  OutDataTypeStr=fixdt(1,32,25)
  Max : MinMax  Function=max
  Min : MinMax
  ABC_SVM : Outport  VectorParamsAs1DForOutWhenUnconnected=off
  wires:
  Add/1 -> Gain/1
  Max/1 -> Add/1
  Min/1 -> Add/2
  Gain/1 -> Add1/2
  ABC/1 -> Add1/1, Max/1, Min/1
  Add1/1 -> ABC_SVM/1

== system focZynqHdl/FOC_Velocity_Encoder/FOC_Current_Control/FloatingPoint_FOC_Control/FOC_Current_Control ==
  note: FOC Current Control
  Reset : Inport  SampleTime=sampleTime.CurrentControl
  Current_Command : Inport  Port=2  OutMin=dataRange.PhaseCurrent.Min  OutMax=dataRange.PhaseCurrent.Max  SampleTime=sampleTime.CurrentControl
  Phase_Current : Inport  Port=3  OutMin=dataRange.PhaseCurrent.Min  OutMax=dataRange.PhaseCurrent.Max  SampleTime=sampleTime.CurrentControl
  Electrical_Position : Inport  Port=4  OutMin=0  OutMax=2*pi  SampleTime=sampleTime.CurrentControl
  Clarke_Transform : Subsystem
  DQ_Current_Control : Subsystem
  Inverse_Clarke_Transform : Subsystem  VariantControl=INVERSE_CLARKE_TRANSFORM
  Inverse_Park_Transform : Subsystem
  Park_Transform : Subsystem
  Sat : Saturate  UpperLimit=dataRange.PhaseVoltage.Max  LowerLimit=dataRange.PhaseVoltage.Min  OutDataTypeStr=Inherit: Inherit via back propagation
  Space_Vector_Modulation : Subsystem  VariantControl=SpaceVectorModulation_JB
  Trigonometric Function : Trigonometry  Operator=sincos
  Phase_Voltage : Outport  SampleTime=sampleTime.CurrentControl  VectorParamsAs1DForOutWhenUnconnected=off
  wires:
  Trigonometric Function/1 -> Inverse_Park_Transform/3(Sin_Coefficient1), Park_Transform/3(Sin_Coefficient1)  "sinCoefficient"
  Trigonometric Function/2 -> Park_Transform/4(Cos_Coefficient1), Inverse_Park_Transform/4(Cos_Coefficient1)  "cosCoefficient"
  Inverse_Clarke_Transform/1(ABC) -> Space_Vector_Modulation/1(ABC)  "abcVoltage"
  Electrical_Position/1 -> Trigonometric Function/1
  Phase_Current/1 -> Clarke_Transform/1(ABC)
  Clarke_Transform/1(Alpha) -> Park_Transform/1(Alpha)  "alphaCurrent"
  Clarke_Transform/2(Beta) -> Park_Transform/2(Beta1)  "betaCurrent"
  Inverse_Park_Transform/1(Alpha) -> Inverse_Clarke_Transform/1(Alpha)  "alphaVoltage"
  Inverse_Park_Transform/2(Beta) -> Inverse_Clarke_Transform/2(Beta)  "betaVoltage"
  Park_Transform/1(D) -> DQ_Current_Control/3(D_Current)  "dCurrent"
  Park_Transform/2(Q) -> DQ_Current_Control/4(Q_Current)  "qCurrent"
  Current_Command/1 -> DQ_Current_Control/2(Q_Command)
  DQ_Current_Control/1(D_Voltage) -> Inverse_Park_Transform/1(D)  "dVoltage"
  DQ_Current_Control/2(Q_Voltage) -> Inverse_Park_Transform/2(Q)  "qVoltage"
  Space_Vector_Modulation/1(ABC_SVM) -> Sat/1  "svmVoltage"
  Sat/1 -> Phase_Voltage/1
  Reset/1 -> DQ_Current_Control/1(Reset)

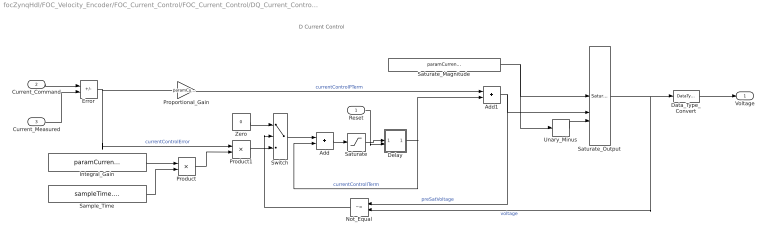
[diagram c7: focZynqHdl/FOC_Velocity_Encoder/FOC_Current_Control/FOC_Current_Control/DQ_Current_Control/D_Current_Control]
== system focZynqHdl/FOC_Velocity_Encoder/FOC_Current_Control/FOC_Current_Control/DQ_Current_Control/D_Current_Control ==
  note: D Current Control
  Reset : Inport
  Current_Command : Inport  Port=2
  Current_Measured : Inport  Port=3
  Add : Sum  OutDataTypeStr=fixdt(1,32,25)
  Add1 : Sum  OutDataTypeStr=fixdt(1,32,19)
  Data_Type_Convert : DataTypeConversion  OutDataTypeStr=fixdt(1,16,11)  RndMeth=Simplest
  Delay : Subsystem
  Error : Sum  Inputs=+-  OutDataTypeStr=fixdt(1,16,9)
  Integral_Gain : Constant  Value=paramCurrentControlI  OutDataTypeStr=fixdt(1,16,3)  SampleTime=-1
  Not_Equal : RelationalOperator  Operator=~=  OutDataTypeStr=boolean
  Product : Product  OutDataTypeStr=fixdt(1,16,15)
  Product1 : Product  OutDataTypeStr=fixdt(1,32,26)
  Proportional_Gain : Gain  Gain=paramCurrentControlP  ParamDataTypeStr=fixdt(1,16,8)  OutDataTypeStr=fixdt(1,32,19)
  Sample_Time : Constant  Value=sampleTime.CurrentControl  OutDataTypeStr=fixdt(1,16,27)  SampleTime=-1
  Saturate : Saturate  UpperLimit=dataRange.DqVoltage.Max  LowerLimit=dataRange.DqVoltage.Min
  Saturate_Magnitude : Constant  Value=paramCurrentControlSatVoltage  OutDataTypeStr=fixdt(1,16,11)  SampleTime=-1
  Saturate_Output : simulink/Discontinuities/Saturation Dynamic  OutMin=[]  OutMax=[]  OutDataTypeStr=Inherit: Same as second input  OutDataType=fixdt(1, 16)  OutScaling=2^-10  DoSatur=off
  Switch : Switch  Criteria=u2 ~= 0  OutDataTypeStr=fixdt(1,32,26)
  Unary_Minus : UnaryMinus
  Zero : Constant  Value=0  OutDataTypeStr=fixdt(1,16,0)  SampleTime=-1
  Voltage : Outport  VectorParamsAs1DForOutWhenUnconnected=off
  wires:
  Data_Type_Convert/1 -> Voltage/1
  Product1/1 -> Switch/3
  Product/1 -> Product1/2
  Sample_Time/1 -> Product/2
  Integral_Gain/1 -> Product/1
  Unary_Minus/1 -> Saturate_Output/3
  Saturate_Magnitude/1 -> Unary_Minus/1, Saturate_Output/1
  Saturate/1 -> Delay/1(In)
  Zero/1 -> Switch/1
  Switch/1 -> Add/1
  Not_Equal/1 -> Switch/2
  Add/1 -> Saturate/1
  Saturate_Output/1 -> Data_Type_Convert/1, Not_Equal/2  "voltage"
  Error/1 -> Product1/1, Proportional_Gain/1  "currentControlError"
  Proportional_Gain/1 -> Add1/1  "currentControlPTerm"
  Current_Command/1 -> Error/1
  Add1/1 -> Saturate_Output/2, Not_Equal/1  "preSatVoltage"
  Delay/1(Out) -> Add1/2, Add/2  "currentControlITerm"
  Current_Measured/1 -> Error/2
  Reset/1 -> Delay/2(Reset1)

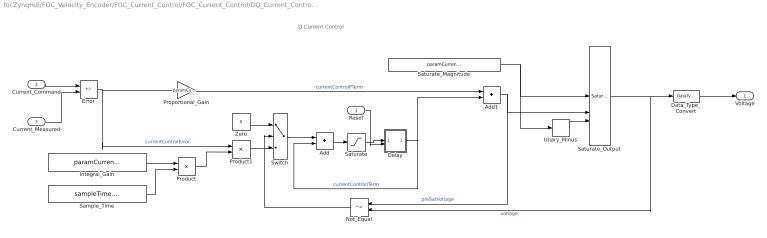
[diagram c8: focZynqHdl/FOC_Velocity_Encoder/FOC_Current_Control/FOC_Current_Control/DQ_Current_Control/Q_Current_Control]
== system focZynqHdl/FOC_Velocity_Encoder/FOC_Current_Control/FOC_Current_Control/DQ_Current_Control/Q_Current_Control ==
  note: Q Current Control
  Reset : Inport
  Current_Command : Inport  Port=2
  Current_Measured : Inport  Port=3
  Add : Sum  OutDataTypeStr=fixdt(1,32,25)
  Add1 : Sum  OutDataTypeStr=fixdt(1,32,18)
  Data_Type_Convert : DataTypeConversion  OutDataTypeStr=fixdt(1,16,11)  RndMeth=Simplest
  Delay : Subsystem
  Error : Sum  Inputs=+-  OutDataTypeStr=fixdt(1,16,9)
  Integral_Gain : Constant  Value=paramCurrentControlI  OutDataTypeStr=fixdt(1,16,3)  SampleTime=-1
  Not_Equal : RelationalOperator  Operator=~=  OutDataTypeStr=boolean
  Product : Product  OutDataTypeStr=fixdt(1,16,15)
  Product1 : Product  OutDataTypeStr=fixdt(1,32,26)
  Proportional_Gain : Gain  Gain=paramCurrentControlP  ParamDataTypeStr=fixdt(1,16,8)  OutDataTypeStr=fixdt(1,32,18)
  Sample_Time : Constant  Value=sampleTime.CurrentControl  OutDataTypeStr=fixdt(1,16,27)  SampleTime=-1
  Saturate : Saturate  UpperLimit=dataRange.DqVoltage.Max  LowerLimit=dataRange.DqVoltage.Min
  Saturate_Magnitude : Constant  Value=paramCurrentControlSatVoltage  OutDataTypeStr=fixdt(1,16,11)  SampleTime=-1
  Saturate_Output : simulink/Discontinuities/Saturation Dynamic  OutMin=[]  OutMax=[]  OutDataTypeStr=Inherit: Same as second input  OutDataType=fixdt(1, 16)  OutScaling=2^-10  DoSatur=off
  Switch : Switch  Criteria=u2 ~= 0  OutDataTypeStr=fixdt(1,32,26)
  Unary_Minus : UnaryMinus
  Zero : Constant  Value=0  OutDataTypeStr=fixdt(1,16,0)  SampleTime=-1
  Voltage : Outport  VectorParamsAs1DForOutWhenUnconnected=off
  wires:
  Data_Type_Convert/1 -> Voltage/1
  Product1/1 -> Switch/3
  Product/1 -> Product1/2
  Sample_Time/1 -> Product/2
  Integral_Gain/1 -> Product/1
  Unary_Minus/1 -> Saturate_Output/3
  Saturate_Magnitude/1 -> Unary_Minus/1, Saturate_Output/1
  Saturate/1 -> Delay/1(In)
  Zero/1 -> Switch/1
  Switch/1 -> Add/1
  Not_Equal/1 -> Switch/2
  Add/1 -> Saturate/1
  Saturate_Output/1 -> Data_Type_Convert/1, Not_Equal/2  "voltage"
  Error/1 -> Product1/1, Proportional_Gain/1  "currentControlError"
  Proportional_Gain/1 -> Add1/1  "currentControlPTerm"
  Current_Command/1 -> Error/1
  Add1/1 -> Saturate_Output/2, Not_Equal/1  "preSatVoltage"
  Delay/1(Out) -> Add1/2, Add/2  "currentControlITerm"
  Current_Measured/1 -> Error/2
  Reset/1 -> Delay/2(Reset1)

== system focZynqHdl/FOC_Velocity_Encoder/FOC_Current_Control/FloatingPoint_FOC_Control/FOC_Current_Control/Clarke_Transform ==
  note: Clarke Transform
  note: Converts balanced three-phase quantities into balanced two-phase quantities. The A and B phases are converted to the direct axis (alpha) component and the quadrature axis (beta) component. The alpha and beta components are still dependent on time and speed.
  ABC : Inport
  A : Selector  IndexMode=Zero-based  InputPortWidth=2  IndexOptions=Index vector (dialog)  Indices=0  OutputSizes=1
  Add : Sum  OutDataTypeStr=Inherit: Inherit via back propagation
  Alpha_Gain : Gain  Gain=1/sqrt(3)  OutDataTypeStr=Inherit: Inherit via back propagation
  B : Selector  IndexMode=Zero-based  InputPortWidth=2  IndexOptions=Index vector (dialog)  Indices=1  OutputSizes=1
  Beta_Gain : Gain  Gain=2/sqrt(3)  OutDataTypeStr=Inherit: Inherit via back propagation
  Alpha : Outport  VectorParamsAs1DForOutWhenUnconnected=off
  Beta : Outport  Port=2  VectorParamsAs1DForOutWhenUnconnected=off
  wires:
  Add/1 -> Beta/1
  B/1 -> Beta_Gain/1
  Beta_Gain/1 -> Add/2
  ABC/1 -> A/1, B/1
  Alpha_Gain/1 -> Add/1
  A/1 -> Alpha_Gain/1, Alpha/1

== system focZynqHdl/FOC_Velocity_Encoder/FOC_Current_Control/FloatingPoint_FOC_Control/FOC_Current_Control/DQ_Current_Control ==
  note: DQ Current Control
  Reset : Inport
  Q_Command : Inport  Port=2  SampleTime=sampleTime.CurrentControl
  D_Current : Inport  Port=3
  Q_Current : Inport  Port=4
  D_Command : Constant  Value=0  OutDataTypeStr=Inherit: Inherit via back propagation  SampleTime=-1
  D_Current_Control : Subsystem
  Q_Current_Control : Subsystem
  Reset1 : InportShadow
  D_Voltage : Outport  VectorParamsAs1DForOutWhenUnconnected=off
  Q_Voltage : Outport  Port=2  VectorParamsAs1DForOutWhenUnconnected=off
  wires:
  Q_Current_Control/1(Voltage) -> Q_Voltage/1
  D_Current_Control/1(Voltage) -> D_Voltage/1
  D_Command/1 -> D_Current_Control/2(Current_Command)
  Q_Command/1 -> Q_Current_Control/2(Current_Command)
  Q_Current/1 -> Q_Current_Control/3(Current_Measured)
  D_Current/1 -> D_Current_Control/3(Current_Measured)
  Reset/1 -> D_Current_Control/1(Reset)
  Reset1/1 -> Q_Current_Control/1(Reset)
